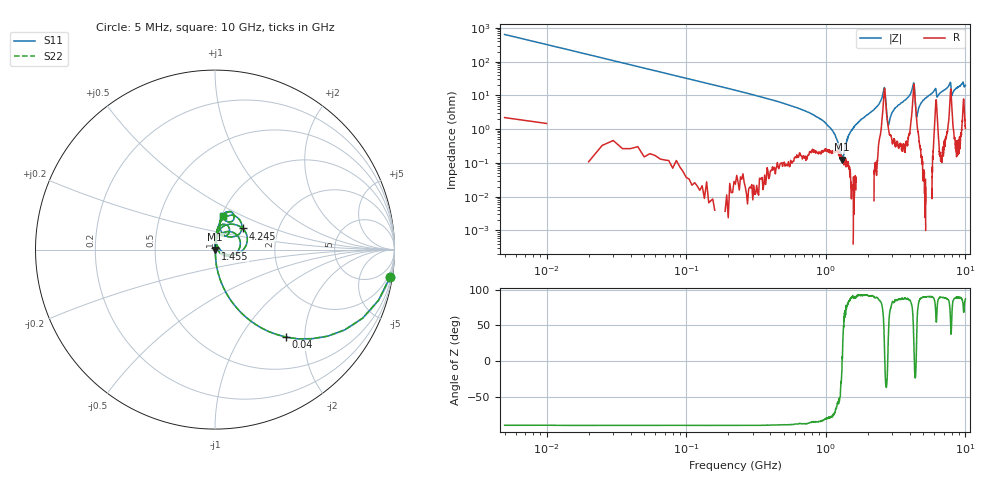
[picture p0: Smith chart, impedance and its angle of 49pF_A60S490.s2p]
! Amotech Co.,Ltd.
! http://www.amotech.co.kr/
! Part Number: A60S490
! These Parameters are Measured in Series Mode Connection
! Operation Temp=25[degC], DC Bias Voltage=0[V]
! Freq. Start=5[MHz] Stop=10[GHz], 2000[Steps]
! Date: Monday, July 13, 2020, 01:42:59
# GHZ S RI R 50.000000
!Freq.(Hz) S11(Real) S11(Imag) S21(Real) S21(Imag) S12(Real) S12(Imag) S22(Real) S22(Imag)
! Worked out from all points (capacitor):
!   2000 points, 5 MHz to 10 GHz, reference 50 ohm
!   read as one part in series: C = 48.9 pF near 55 MHz
!   lowest |Z| = 124 mohm at 1.3 GHz (marker M1)
!   series resonance near 1.308 GHz, so ESL is about 300 pH
!   S11 on the Smith chart (normalised r, x): 5 MHz: 1, -13; 40 MHz: 1.01, -1.62; 1.455 GHz: 1.00, +0.01; 4.245 GHz: 1.32, +0.32; 10 GHz: 1.02, +0.40
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0.005  0.9757 -0.1524  0.0243 0.1524  0.0243 0.1524  0.9757 -0.1524
0.04  0.3967 -0.4876  0.6033 0.4876  0.6033 0.4876  0.3967 -0.4876
0.095  0.1046 -0.3053  0.8954 0.3053  0.8954 0.3053  0.1046 -0.3053
0.18  0.031 -0.1734  0.969 0.1734  0.969 0.1734  0.031 -0.1734
1.04  0.00229 -0.0122  0.9977 0.0122  0.9977 0.0122  0.00229 -0.0122
1.3  0.00119 -0.000329  0.9988 0.000329  0.9988 0.000329  0.00119 -0.000329
1.455  0.000907 0.00653  0.9991 -0.00653  0.9991 -0.00653  0.000907 0.00653
1.675  0.000143 0.0147  0.9999 -0.0147  0.9999 -0.0147  0.000143 0.0147
2.37  0.00491 0.0505  0.9951 -0.0505  0.9951 -0.0505  0.00491 0.0505
2.61  0.1132 0.0886  0.8868 -0.0886  0.8868 -0.0886  0.1132 0.0886
2.81  0.0102 0.00807  0.9898 -0.00807  0.9898 -0.00807  0.0102 0.00807
3.34  0.006 0.0524  0.994 -0.0524  0.994 -0.0524  0.006 0.0524
4.245  0.1541 0.1176  0.8459 -0.1176  0.8459 -0.1176  0.1541 0.1176
4.48  0.018 0.0136  0.982 -0.0136  0.982 -0.0136  0.018 0.0136
5.005  0.00563 0.0722  0.9944 -0.0722  0.9944 -0.0722  0.00563 0.0722
6.085  0.0525 0.1414  0.9475 -0.1414  0.9475 -0.1414  0.0525 0.1414
6.265  0.0339 0.0794  0.9661 -0.0794  0.9661 -0.0794  0.0339 0.0794
6.67  0.0163 0.1212  0.9837 -0.1212  0.9837 -0.1212  0.0163 0.1212
7.77  0.1128 0.1868  0.8872 -0.1868  0.8872 -0.1868  0.1128 0.1868
7.99  0.0517 0.0787  0.9483 -0.0787  0.9483 -0.0787  0.0517 0.0787
8.335  0.0246 0.1378  0.9754 -0.1378  0.9754 -0.1378  0.0246 0.1378
10  0.0473 0.1876  0.9527 -0.1876  0.9527 -0.1876  0.0473 0.1876
